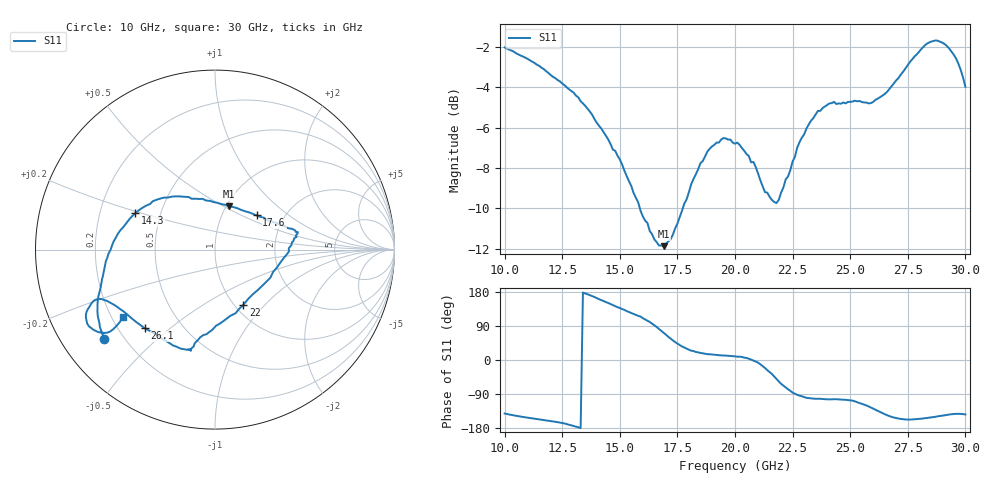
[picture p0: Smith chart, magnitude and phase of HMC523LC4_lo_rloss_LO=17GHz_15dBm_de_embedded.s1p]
!Hittite Microwave Corporation
!20 Alpha Rd
!Chelmsford, MA 01824
!Tel: 978-250-3343
!Fax: 978-250-3373
!Device: HMC523LC4, 10-30 GHz, GaAs MMIC Double-Balanced Mixer
!Misc: LO Return Loss with LO at 15 dBm, Room
# MHZ S MA R 50
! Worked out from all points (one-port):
!   201 points, 10 GHz to 30 GHz, reference 50 ohm
!   lowest |S11| = -11.9 dB at 16.9 GHz (marker M1), VSWR 1.68, Z = 51.6 + j26.7 ohm
!   |S11| at or under -10 dB: 15.87 GHz to 17.73 GHz (1.862 GHz wide, 11.1 % of centre)
!   S11 on the Smith chart (normalised r, x): 10 GHz: 0.13, -0.35; 14.3 GHz: 0.36, +0.19; 17.6 GHz: 1.46, +0.61; 22 GHz: 1.09, -0.77; 26.1 GHz: 0.31, -0.41; 30 GHz: 0.25, -0.31
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10000  0.791 -141.1
11000  0.741 -152.1
12500  0.644 -166.3
13500  0.567 175.5
14300  0.488 155.4
15000  0.418 137.3
16300  0.278 100.3
16900  0.255 71.8
17500  0.29 43.5
17600  0.301 39.3
18800  0.437 15.4
19500  0.472 11.9
20000  0.457 9.6
20500  0.431 5.4
20900  0.4 -4.1
21600  0.332 -36.8
22000  0.346 -62.9
22500  0.413 -86.2
23300  0.521 -101.3
24300  0.58 -103.5
25000  0.58 -106.4
26100  0.587 -131.7
26800  0.634 -150.2
27500  0.715 -157.2
28200  0.796 -154.1
28700  0.823 -149.9
29500  0.758 -142.4
30000  0.632 -143.8
